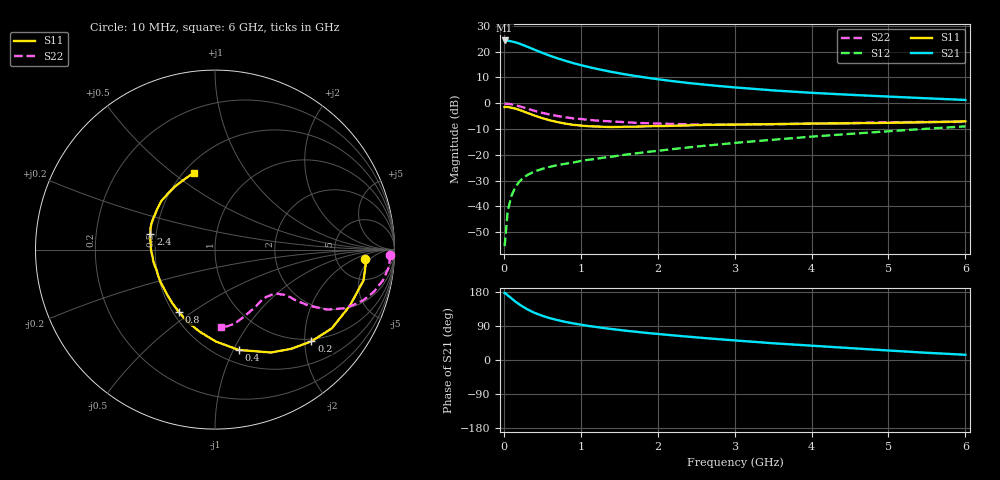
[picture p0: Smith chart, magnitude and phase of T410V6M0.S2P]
! Infineon Technologies  Discrete & RF Semiconductors
! BFR182T
! Si NPN RF Bipolar Junction Transistor in SC75
! VCE = 10 V  IC = 6 mA
! Common Emitter S-Parameters:  October  1999
# GHz  S  MA  R  50
!  f  S11  S21  S12  S22
! GHz  MAG  ANG  MAG  ANG  MAG  ANG  MAG  ANG
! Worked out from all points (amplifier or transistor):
!   36 points, 10 MHz to 6 GHz, reference 50 ohm
!   highest |S21| = 24.3 dB at 10 MHz (marker M1)
!   |S21| within 3 dB of that: start of sweep to 351.3 MHz
!   unconditionally stable (mu >= 1): 1.386 GHz to 4.19 GHz
!   at 250 MHz: K = 0.31, MSG = 25.8 dB, |S12| = -29.0 dB
!   at 1.4 GHz: K = 1.00, MAG = 16.0 dB, |S12| = -20.8 dB
!   at 6 GHz: K = 0.86, MSG = 5.1 dB, |S12| = -9.0 dB
!   S11 on the Smith chart (normalised r, x): 10 MHz: 10, -3; 200 MHz: 0.95, -2.15; 400 MHz: 0.63, -1.05; 800 MHz: 0.54, -0.44; 2.4 GHz: 0.46, +0.10; 6 GHz: 0.56, +0.60
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0.01  0.8392 -3.4  16.38 176.8  0.0017 82.8  0.9763 -1.8
0.02  0.8459 -3.4  16.23 176.2  0.0024 90.0  0.9742 -2.1
0.05  0.845 -11.7  16.22 170.8  0.0081 85.1  0.9758 -5.4
0.1  0.8139 -22.6  15.72 162.6  0.0162 79.6  0.9509 -10.4
0.15  0.7849 -34.0  15.08 154.2  0.0238 72.3  0.9148 -15.0
0.2  0.7415 -43.6  14.27 146.9  0.0301 69.7  0.8747 -18.7
0.25  0.6965 -52.6  13.34 140.4  0.0354 64.8  0.8296 -21.9
0.3  0.6523 -61.5  12.46 134.4  0.0401 62.6  0.7885 -24.5
0.4  0.5743 -76.7  10.83 124.4  0.0477 58.3  0.7096 -28.1
0.5  0.5121 -89.5  9.428 116.7  0.0533 56.5  0.6491 -29.7
0.6  0.4642 -100.9  8.277 110.3  0.0586 54.9  0.6009 -31.0
0.7  0.4293 -111.2  7.364 105.1  0.0633 54.7  0.5631 -31.6
0.8  0.4014 -120.1  6.62 100.6  0.0671 54.5  0.5333 -32.1
0.9  0.3811 -128.8  5.975 96.7  0.0707 54.9  0.5085 -32.3
1.1  0.3569 -143.4  5.024 89.9  0.08 55.7  0.4756 -32.9
1.6  0.3502 -169.9  3.571 77.0  0.1014 58.1  0.425 -35.2
2.2  0.3648 171.0  2.665 65.0  0.1292 60.5  0.397 -40.4
2.4  0.3711 166.1  2.459 61.5  0.139 60.7  0.3891 -42.6
3.5  0.3926 145.5  1.767 44.2  0.1958 60.2  0.3914 -55.4
4.5  0.4069 131.0  1.453 31.4  0.2541 57.3  0.4119 -69.0
5.5  0.4274 113.4  1.242 19.0  0.3199 53.0  0.4328 -80.9
6  0.4445 105.1  1.154 13.8  0.3554 49.9  0.4333 -85.9
